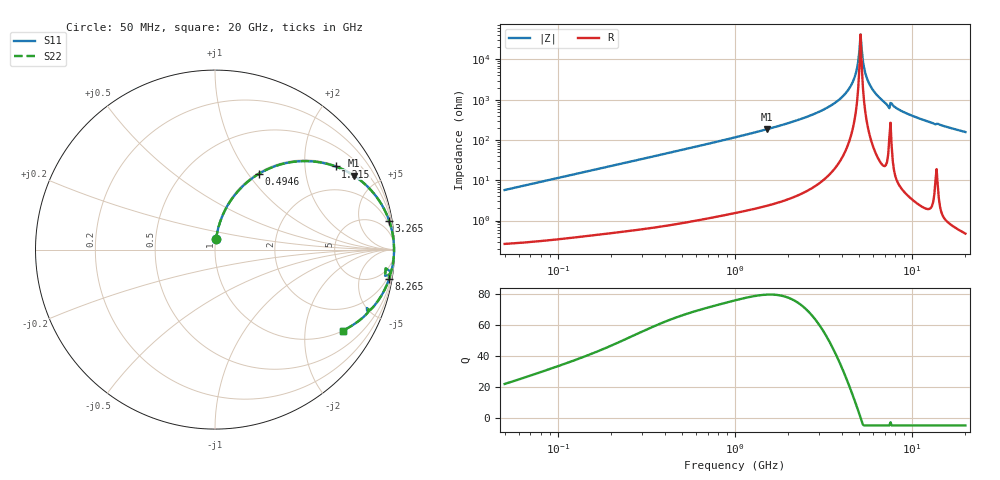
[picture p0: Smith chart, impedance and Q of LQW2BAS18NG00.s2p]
!Murata Part Number: LQW2BAS18NG00
!These Parameters are Measured in Series Mode Connection
!  o--[Z]--o
!Port1  Port2
!  o-------o
!Freq. Start=50[MHz] Stop=20[GHz], 401[Steps]
# Hz S RI R 50
!Freq.(Hz) S11(Real) S11(Imag) S21(Real) S21(Imag) S12(Real) S12(Imag) S22(Real) S22(Imag)
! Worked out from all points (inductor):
!   401 points, 50 MHz to 20 GHz, reference 50 ohm
!   read as one part in series: L = 18.2 nH near 51.52 MHz
!   highest Q = 79.5 at 1.521 GHz (marker M1), where L = 19.5 nH
!   self-resonance near 5.118 GHz
!   S11 on the Smith chart (normalised r, x): 50 MHz: 1.01, +0.11; 494.6 MHz: 1.02, +1.12; 1.215 GHz: 1.04, +2.87; 3.265 GHz: 1, +12; 8.265 GHz: 1, -12; 20 GHz: 1.01, -3.16
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5e7  0.00587 0.0568  0.9941 -0.0568  0.9941 -0.0568  0.00587 0.0568
1.364002e8  0.0272 0.1502  0.9728 -0.1502  0.9728 -0.1502  0.0272 0.1502
3.721004e8  0.1547 0.3535  0.8453 -0.3535  0.8453 -0.3535  0.1547 0.3535
4.946044e8  0.2427 0.4212  0.7573 -0.4212  0.7573 -0.4212  0.2427 0.4212
1e9  0.5737 0.488  0.4263 -0.488  0.4263 -0.488  0.5737 0.488
1.214974e9  0.6718 0.4632  0.3282 -0.4632  0.3282 -0.4632  0.6718 0.4632
1.521052e9  0.7729 0.4127  0.2271 -0.4127  0.2271 -0.4127  0.7729 0.4127
2.728004e9  0.9442 0.2221  0.0558 -0.2221  0.0558 -0.2221  0.9442 0.2221
3.265178e9  0.9711 0.1584  0.0289 -0.1584  0.0289 -0.1584  0.9711 0.1584
3.967106e9  0.9892 0.0896  0.0108 -0.0896  0.0108 -0.0896  0.9892 0.0896
4.472136e9  0.9952 0.0475  0.00479 -0.0475  0.00479 -0.0475  0.9952 0.0475
4.748272e9  0.9968 0.0265  0.00316 -0.0265  0.00316 -0.0265  0.9968 0.0265
4.966507e9  0.9975 0.0107  0.00253 -0.0107  0.00253 -0.0107  0.9975 0.0107
5.117541e9  0.9976 0.000202  0.00238 -0.000202  0.00238 -0.000202  0.9976 0.000202
5.273168e9  0.9975 -0.0103  0.00247 0.0103  0.00247 0.0103  0.9975 -0.0103
5.515528e9  0.997 -0.0262  0.00302 0.0262  0.00302 0.0262  0.997 -0.0262
5.856089e9  0.9954 -0.0475  0.00458 0.0475  0.00458 0.0475  0.9954 -0.0475
6.601595e9  0.9891 -0.0912  0.0109 0.0912  0.0109 0.0912  0.9891 -0.0912
7.442007e9  0.9476 -0.1462  0.0524 0.1462  0.0524 0.1462  0.9476 -0.1462
8.264682e9  0.9703 -0.1622  0.0297 0.1622  0.0297 0.1622  0.9703 -0.1622
1.314879e10  0.8679 -0.3332  0.1321 0.3332  0.1321 0.3332  0.8679 -0.3332
2e10  0.7131 -0.4508  0.2869 0.4508  0.2869 0.4508  0.7131 -0.4508
